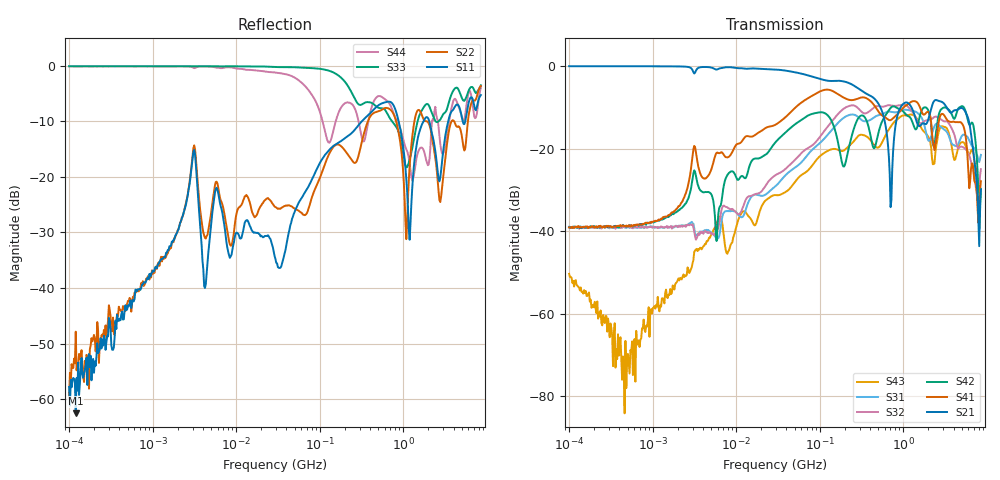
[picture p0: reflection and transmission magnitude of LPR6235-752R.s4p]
# MHz S MA R 50
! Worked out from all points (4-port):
!   498 points, 100 kHz to 8.5 GHz, reference 50 ohm
!   strongest paths, dB at 100 kHz, 1.698 MHz, 29.49 MHz, 500.7 MHz, 8.5 GHz:
!     S21: -0.1, -0.1, -0.8, -9.0, -29.9
!     S41: -39.1, -35.5, -14.2, -10.9, -27.9
!     S42: -39.1, -35.9, -18.5, -16.5, -29.7
!     S32: -39.2, -39.4, -26.5, -9.7, -25.0
!     S31: -39.0, -39.0, -29.1, -11.9, -21.5
!     S43: -50.4, -55.1, -31.3, -19.8, -31.1
!   lowest |S11| = -62.6 dB at 120 kHz (marker M1), VSWR 1.00, Z = 50 + j0.06 ohm
!   |S11| at or under -10 dB: start of sweep to 318.3 MHz; 882.2 MHz to 1.746 GHz (864.2 MHz wide, 65.8 % of centre); 2.054 GHz to 3.452 GHz (1.399 GHz wide, 50.8 % of centre)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
0.1  0.001289 -6.0  0.9942 -0.1  0.01126 179.0  0.01106 6.3
     0.9942 -0.1  0.001017 114.3  0.01103 2.2  0.01112 177.1
     0.01126 179.0  0.01103 2.2  0.9927 0.2  0.00303 -87.1
     0.01106 6.3  0.01112 177.1  0.00303 -87.1  0.9931 0.0
0.1200457  0.0007447 53.7  0.9938 -0.1  0.01106 178.9  0.01132 6.3
           0.9938 -0.1  0.004044 87.1  0.01133 2.6  0.01125 174.4
           0.01106 178.9  0.01133 2.6  0.9929 0.1  0.002545 -87.5
           0.01132 6.3  0.01125 174.4  0.002545 -87.5  0.9929 -0.0
0.4725499  0.007005 87.1  0.9948 -0.6  0.01099 177.5  0.01148 19.8
           0.9948 -0.6  0.006211 96.1  0.01121 2.7  0.0114 158.6
           0.01099 177.5  0.01121 2.7  0.9938 -0.1  0.0004669 21.2
           0.01148 19.8  0.0114 158.6  0.0004669 21.2  0.9919 -0.5
118.7648  0.1618 162.5  0.6685 -38.7  0.1388 58.8  0.5168 -2.5
          0.6685 -38.7  0.1384 49.4  0.1731 53.9  0.2633 -23.1
          0.1388 58.8  0.1731 53.9  0.921 -39.8  0.09115 37.8
          0.5168 -2.5  0.2633 -23.1  0.09115 37.8  0.2363 -57.8
705.2109  0.4731 -100.2  0.01948 -150.9  0.2795 -83.9  0.2209 -98.4
          0.01948 -150.9  0.4023 -122.7  0.3334 -88.3  0.3103 -67.8
          0.2795 -83.9  0.3334 -88.3  0.3303 -137.3  0.1831 -49.8
          0.2209 -98.4  0.3103 -67.8  0.1831 -49.8  0.4395 -132.6
4383.155  0.4492 -169.2  0.2932 140.6  0.1075 143.5  0.209 130.0
          0.2932 140.6  0.2834 -154.7  0.1096 119.8  0.2768 142.0
          0.1075 143.5  0.1096 119.8  0.6375 178.4  0.08794 172.1
          0.209 130.0  0.2768 142.0  0.08794 172.1  0.4743 -173.8
8500  0.5464 -44.7  0.03211 57.3  0.08379 13.3  0.04018 58.8
      0.03211 57.3  0.6585 -34.0  0.05627 59.8  0.0326 14.6
      0.08379 13.3  0.05627 59.8  0.6679 -35.3  0.02771 56.5
      0.04018 58.8  0.0326 14.6  0.02771 56.5  0.6307 -37.6
